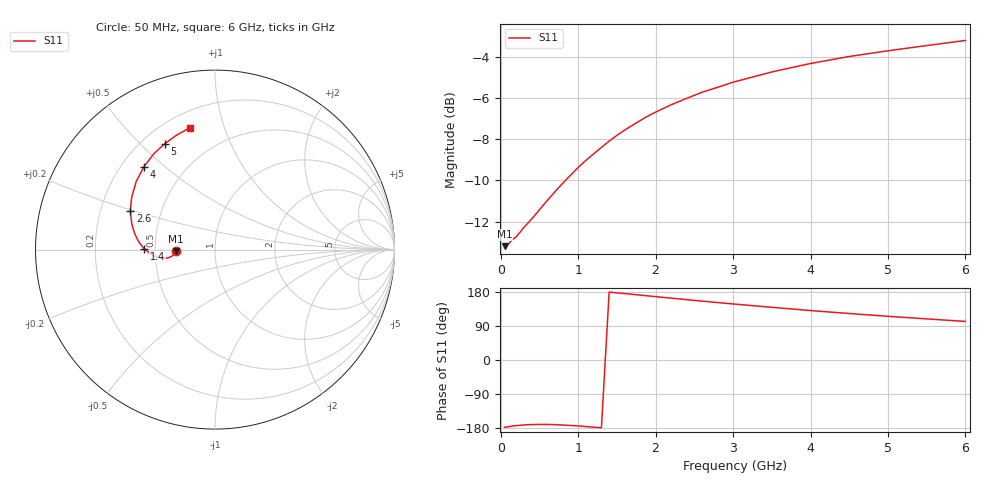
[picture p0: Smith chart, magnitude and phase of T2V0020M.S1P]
! SIEMENS Discrete & RF Semiconductors
! BAS70-04W
! Si Schottky Diode in SOT323
! IF = 20 mA
! S-Parameters:  November  1997
# GHz  S  MA  R  50
!  f  S11
! GHz  MAG  ANG
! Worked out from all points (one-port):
!   34 points, 50 MHz to 6 GHz, reference 50 ohm
!   lowest |S11| = -13.2 dB at 50 MHz (marker M1), VSWR 1.56, Z = 32.1 - j0.643 ohm
!   |S11| at or under -10 dB: start of sweep to 836 MHz
!   S11 on the Smith chart (normalised r, x): 50 MHz: 0.64, -0.01; 1.4 GHz: 0.43, +0.01; 2.6 GHz: 0.33, +0.20; 4 GHz: 0.29, +0.43; 5 GHz: 0.29, +0.60; 6 GHz: 0.30, +0.77
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0.05  0.2189 -177.5
0.1  0.2216 -176.1
0.15  0.227 -174.3
0.2  0.2307 -173.1
0.25  0.2367 -172.4
0.3  0.2432 -171.3
0.4  0.2548 -170.5
0.5  0.2684 -170.0
0.6  0.2824 -170.0
0.7  0.2969 -170.6
0.8  0.3113 -171.6
1  0.34 -173.9
1.1  0.3539 -175.6
1.3  0.3804 -178.9
1.4  0.3941 179.2
1.6  0.4191 175.4
1.8  0.4421 171.3
2  0.4636 167.2
2.2  0.483 163.3
2.4  0.5005 159.2
2.6  0.5182 155.4
3  0.5481 147.9
3.5  0.5805 139.1
4  0.6085 130.5
4.5  0.6329 122.7
5  0.6534 115.3
5.5  0.6728 108.5
6  0.6923 101.8
